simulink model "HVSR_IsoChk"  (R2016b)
settings: Solver=VariableStepAuto  StartTime=0.0  StopTime=10.0  RelTol=1e-3
undefined symbols (not defined in the file or in its folder): bin2dec, enmActv, enmBmsMode, enmCctErr, enmSWSta, HVSR_bIsoResShieldCal, HVSR_bSw1EnaByMnl_C, HVSR_bSw2EnaByMnl_C, HVSR_bSw3EnaByMnl_C, HVSR_bSwEnaByMnl_C, HVSR_bVldEnaByMnl_C, HVSR_cntIsoChkCnfDiag_C, HVSR_cntIsoChkCnfLv1Diag_C, HVSR_cntIsoChkDiag_CW, HVSR_cntPwrDown_C, HVSR_cofPosVoltfilter_C, HVSR_cofResGain_C, HVSR_deltInsRes_C, HVSR_InsResCtrlSw_C, HVSR_kSlopeVal_C, HVSR_numBgnTimeCnt_C, HVSR_numCycleTimeCnt_C, HVSR_numIsoCnst_C, HVSR_numSlopeCnfrm_C, HVSR_ResFirstCtrlSw_C, HVSR_resIsoFaultLvl1Thres_C, HVSR_resIsoFaultLvl2Thres_C, HVSR_ResR1_C, HVSR_ResR2_C, HVSR_ResR3_C, HVSR_resRstnUpLim_C, HVSR_rIsoCnfHysDiag_C, HVSR_rIsoCnfHysLv1Diag_C, HVSR_stBMSModeLvl_C, HVSR_tiChkFilteTime_C, HVSR_tiIsoChkCycl_T, HVSR_tiIsoChkDebounce_C, HVSR_tiIsoVldChkDebounce_C, HVSR_tiTaskTime_C, HVSR_tiVoltDiffThres_C, HVSR_uBattVoltRngHi_C, HVSR_uBattVoltRngLo_C, HVSR_uIsoKVoltThres_C, HVSR_uIsoPosVoltFilter_C, HVSR_uIsoVoltThres_C
libraries: simulink x78
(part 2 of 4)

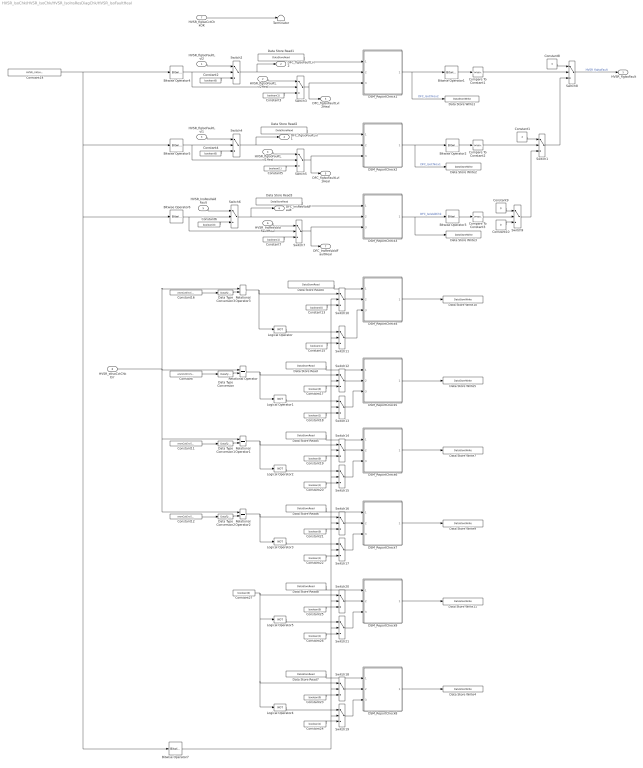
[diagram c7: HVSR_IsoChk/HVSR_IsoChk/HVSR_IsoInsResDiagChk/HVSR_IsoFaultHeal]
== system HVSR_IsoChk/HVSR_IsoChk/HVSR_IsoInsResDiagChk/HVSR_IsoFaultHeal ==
  HVSR_flgIsoFaultLvl2 : Inport
  HVSR_flgIsoFaultLvl2Heal : Inport  Port=2
  HVSR_flgIsoFaultLvl1 : Inport  Port=3
  HVSR_flgIsoFaultLvl1Heal : Inport  Port=4
  HVSR_InsResValdFault : Inport  Port=5
  HVSR_InsResValdFaultHeal : Inport  Port=6
  HVSR_flgIsoCctChkOK : Inport  Port=7
  HVSR_stIsoCctChkErr : Inport  Port=8
  Bitwise Operator1 : simulink/Logic and Bit Operations/Bitwise Operator  logicop=AND  UseBitMask=on  BitMask=bin2dec('00011000')  BitMaskRealWorld=Stored Integer
  Bitwise Operator2 : simulink/Logic and Bit Operations/Bitwise Operator  logicop=AND  UseBitMask=on  BitMask=bin2dec('00011000')  BitMaskRealWorld=Stored Integer
  Bitwise Operator3 : simulink/Logic and Bit Operations/Bitwise Operator  logicop=AND  UseBitMask=on  BitMask=bin2dec('00011000')  BitMaskRealWorld=Stored Integer
  Bitwise Operator4 : simulink/Logic and Bit Operations/Bitwise Operator  logicop=AND  UseBitMask=on  BitMask=bin2dec('00000001')  BitMaskRealWorld=Stored Integer
  Bitwise Operator5 : simulink/Logic and Bit Operations/Bitwise Operator  logicop=AND  UseBitMask=on  BitMask=bin2dec('00000010')  BitMaskRealWorld=Stored Integer
  Bitwise Operator6 : simulink/Logic and Bit Operations/Bitwise Operator  logicop=AND  UseBitMask=on  BitMask=bin2dec('00000100')  BitMaskRealWorld=Stored Integer
  Bitwise Operator7 : simulink/Logic and Bit Operations/Bitwise Operator  logicop=AND  UseBitMask=on  BitMask=bin2dec('00001000')  BitMaskRealWorld=Stored Integer
  Compare To Constant1 : simulink/Logic and Bit Operations/Compare To Constant  relop===  const=24  OutDataTypeStr=boolean
  Compare To Constant2 : simulink/Logic and Bit Operations/Compare To Constant  relop===  const=24  OutDataTypeStr=boolean
  Compare To Constant3 : simulink/Logic and Bit Operations/Compare To Constant  relop===  const=24  OutDataTypeStr=boolean
  Constant : Constant  Value=enmCctErr.S1ERR  OutDataTypeStr=Enum: enmCctErr
  Constant1 : Constant  Value=2  OutDataTypeStr=uint8
  Constant10 : Constant  Value=0  OutDataTypeStr=uint8
  Constant11 : Constant  Value=enmCctErr.S2ERR  OutDataTypeStr=Enum: enmCctErr
  Constant12 : Constant  Value=enmCctErr.S3ERR  OutDataTypeStr=Enum: enmCctErr
  Constant{2,4,6,13,17,19,21,23,25,27} (10 alike) : Constant  Value=boolean(0)
  Constant14 : Constant  Value=HVSR_cntIsoChkDiag_CW
  Constant{3,5,7,15,18,20,22,24,26} (9 alike) : Constant  Value=boolean(1)
  Constant16 : Constant  Value=enmCctErr.CCTCLS  OutDataTypeStr=Enum: enmCctErr
  Constant8 : Constant  Value=3  OutDataTypeStr=uint8
  Constant9 : Constant  Value=0  OutDataTypeStr=uint8
  DSM_ReportCheck1 : Subsystem  TreatAsAtomicUnit=on  RTWFcnName=DSM_ReportCheck  RTWFileName=SrvLib
  DSM_ReportCheck2 : Subsystem  TreatAsAtomicUnit=on  RTWFcnName=DSM_ReportCheck  RTWFileName=SrvLib
  DSM_ReportCheck3 : Subsystem  TreatAsAtomicUnit=on  RTWFcnName=DSM_ReportCheck  RTWFileName=SrvLib
  DSM_ReportCheck4 : Subsystem  TreatAsAtomicUnit=on  RTWFcnName=DSM_ReportCheck  RTWFileName=SrvLib
  DSM_ReportCheck5 : Subsystem  TreatAsAtomicUnit=on  RTWFcnName=DSM_ReportCheck  RTWFileName=SrvLib
  DSM_ReportCheck6 : Subsystem  TreatAsAtomicUnit=on  RTWFcnName=DSM_ReportCheck  RTWFileName=SrvLib
  DSM_ReportCheck7 : Subsystem  TreatAsAtomicUnit=on  RTWFcnName=DSM_ReportCheck  RTWFileName=SrvLib
  DSM_ReportCheck8 : Subsystem  TreatAsAtomicUnit=on  RTWFcnName=DSM_ReportCheck  RTWFileName=SrvLib
  DSM_ReportCheck9 : Subsystem  TreatAsAtomicUnit=on  RTWFcnName=DSM_ReportCheck  RTWFileName=SrvLib
  Data Store Read : DataStoreRead  DataStoreName=DFC_IsoS1SwStuckOpen
  Data Store Read1 : DataStoreRead  DataStoreName=DFC_IsoChkLv2
  Data Store Read2 : DataStoreRead  DataStoreName=DFC_IsoChkLv1
  Data Store Read3 : DataStoreRead  DataStoreName=DFC_InsResValdFault
  Data Store Read4 : DataStoreRead  DataStoreName=DFC_IsoS3SwStuckClsd
  Data Store Read5 : DataStoreRead  DataStoreName=DFC_IsoS2SwStuckOpen
  Data Store Read6 : DataStoreRead  DataStoreName=DFC_IsoS3SwStuckOpen
  Data Store Read7 : DataStoreRead  DataStoreName=DFC_IsoS1SwStuckClsd
  Data Store Read8 : DataStoreRead  DataStoreName=DFC_IsoS2SwStuckClsd
  Data Store Write1 : DataStoreWrite  DataStoreName=DFC_IsoChkLv2
  Data Store Write10 : DataStoreWrite  DataStoreName=DFC_IsoS3SwStuckClsd
  Data Store Write11 : DataStoreWrite  DataStoreName=DFC_IsoS2SwStuckClsd
  Data Store Write2 : DataStoreWrite  DataStoreName=DFC_IsoChkLv1
  Data Store Write3 : DataStoreWrite  DataStoreName=DFC_InsResValdFault
  Data Store Write4 : DataStoreWrite  DataStoreName=DFC_IsoS1SwStuckClsd
  Data Store Write5 : DataStoreWrite  DataStoreName=DFC_IsoS1SwStuckOpen
  Data Store Write7 : DataStoreWrite  DataStoreName=DFC_IsoS2SwStuckOpen
  Data Store Write9 : DataStoreWrite  DataStoreName=DFC_IsoS3SwStuckOpen
  Data Type Conversion{,1..3} (4 alike) : DataTypeConversion  OutDataTypeStr=uint8
  Logical Operator{,1..5} (6 alike) : Logic  Operator=NOT  AllPortsSameDT=off  OutDataTypeStr=boolean
  Relational Operator{,1..3} (4 alike) : RelationalOperator  Operator===  OutDataTypeStr=boolean  RndMeth=Simplest
  Switch{1..21} (21 alike) : Switch  Criteria=u2 ~= 0
  Terminator : Terminator
  " HVSR_flgIsoFault" : Outport
  DFC_flgIsoFaultLvl2 : Outport  Port=2
  DFC_flgIsoFaultLvl2Heal : Outport  Port=3
  DFC_flgIsoFaultLvl1 : Outport  Port=4
  DFC_flgIsoFaultLvl1Heal : Outport  Port=5
  DFC_InsResValdFault : Outport  Port=6
  DFC_InsResValdFaultHeal : Outport  Port=7
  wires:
  Constant14/1 -> Bitwise Operator4/1, Bitwise Operator5/1, Bitwise Operator6/1, Bitwise Operator7/1
  DSM_ReportCheck1/1(Dfc_id) -> Data Store Write1/1, Bitwise Operator1/1  "DFC_IsoChkLv2"
  DSM_ReportCheck2/1(Dfc_id) -> Data Store Write2/1, Bitwise Operator2/1  "DFC_IsoChkLv1"
  Bitwise Operator2/1 -> Compare To Constant2/1
  Bitwise Operator1/1 -> Compare To Constant1/1
  DSM_ReportCheck3/1(Dfc_id) -> Bitwise Operator3/1, Data Store Write3/1  "DFC_IsoValdChk"
  Data Store Read2/1 -> DSM_ReportCheck2/1(Dfc_id_nv)
  Switch8/1 -> " HVSR_flgIsoFault"/1  "HVSR_flgIsoFault"
  Data Store Read3/1 -> DSM_ReportCheck3/1(Dfc_id_nv)
  Data Store Read1/1 -> DSM_ReportCheck1/1(Dfc_id_nv)
  Switch6/1 -> DFC_InsResValdFault/1, DSM_ReportCheck3/2(Err)
  Switch4/1 -> DFC_flgIsoFaultLvl1/1, DSM_ReportCheck2/2(Err)
  Switch3/1 -> DFC_flgIsoFaultLvl2Heal/1, DSM_ReportCheck1/3(Heal)
  Switch2/1 -> DFC_flgIsoFaultLvl2/1, DSM_ReportCheck1/2(Err)
  Switch7/1 -> DFC_InsResValdFaultHeal/1, DSM_ReportCheck3/3(Heal)
  Switch5/1 -> DFC_flgIsoFaultLvl1Heal/1, DSM_ReportCheck2/3(Heal)
  Constant2/1 -> Switch2/3
  Bitwise Operator4/1 -> Switch3/2, Switch2/2
  HVSR_flgIsoFaultLvl2/1 -> Switch2/1
  Constant3/1 -> Switch3/3
  HVSR_flgIsoFaultLvl2Heal/1 -> Switch3/1
  Constant4/1 -> Switch4/3
  Constant5/1 -> Switch5/3
  HVSR_flgIsoFaultLvl1/1 -> Switch4/1
  Bitwise Operator5/1 -> Switch5/2, Switch4/2
  HVSR_flgIsoFaultLvl1Heal/1 -> Switch5/1
  Constant6/1 -> Switch6/3
  Bitwise Operator6/1 -> Switch7/2, Switch6/2
  HVSR_InsResValdFault/1 -> Switch6/1
  Constant7/1 -> Switch7/3
  HVSR_InsResValdFaultHeal/1 -> Switch7/1
  Compare To Constant1/1 -> Switch8/2
  Compare To Constant2/1 -> Switch1/2
  Switch9/1 -> Switch1/3
  Constant1/1 -> Switch1/1
  Constant8/1 -> Switch8/1
  Switch1/1 -> Switch8/3
  Bitwise Operator3/1 -> Compare To Constant3/1
  Compare To Constant3/1 -> Switch9/2
  Constant9/1 -> Switch9/1
  Constant10/1 -> Switch9/3
  DSM_ReportCheck4/1(Dfc_id) -> Data Store Write10/1
  Data Store Read4/1 -> DSM_ReportCheck4/1(Dfc_id_nv)
  Relational Operator3/1 -> Logical Operator/1, Switch10/1
  Constant13/1 -> Switch10/3
  Constant15/1 -> Switch11/3
  Logical Operator/1 -> Switch11/1
  Switch11/1 -> DSM_ReportCheck4/3(Heal)
  Switch10/1 -> DSM_ReportCheck4/2(Err)
  Constant/1 -> Data Type Conversion/1
  Data Type Conversion/1 -> Relational Operator/2
  Constant11/1 -> Data Type Conversion1/1
  Data Type Conversion1/1 -> Relational Operator1/2
  Constant12/1 -> Data Type Conversion2/1
  Data Type Conversion2/1 -> Relational Operator2/2
  HVSR_stIsoCctChkErr/1 -> Relational Operator3/1, Relational Operator2/1, Relational Operator1/1, Relational Operator/1
  Constant16/1 -> Data Type Conversion3/1
  Data Type Conversion3/1 -> Relational Operator3/2
  DSM_ReportCheck5/1(Dfc_id) -> Data Store Write5/1
  Data Store Read/1 -> DSM_ReportCheck5/1(Dfc_id_nv)
  Switch12/1 -> DSM_ReportCheck5/2(Err)
  Relational Operator/1 -> Logical Operator1/1, Switch12/1
  Constant17/1 -> Switch12/3
  Switch13/1 -> DSM_ReportCheck5/3(Heal)
  Logical Operator1/1 -> Switch13/1
  Constant18/1 -> Switch13/3
  DSM_ReportCheck6/1(Dfc_id) -> Data Store Write7/1
  Data Store Read5/1 -> DSM_ReportCheck6/1(Dfc_id_nv)
  Switch14/1 -> DSM_ReportCheck6/2(Err)
  Relational Operator1/1 -> Logical Operator2/1, Switch14/1
  Constant19/1 -> Switch14/3
  Switch15/1 -> DSM_ReportCheck6/3(Heal)
  Logical Operator2/1 -> Switch15/1
  DSM_ReportCheck7/1(Dfc_id) -> Data Store Write9/1
  Data Store Read6/1 -> DSM_ReportCheck7/1(Dfc_id_nv)
  Switch16/1 -> DSM_ReportCheck7/2(Err)
  Relational Operator2/1 -> Logical Operator3/1, Switch16/1
  Constant21/1 -> Switch16/3
  Switch17/1 -> DSM_ReportCheck7/3(Heal)
  Logical Operator3/1 -> Switch17/1
  Constant20/1 -> Switch15/3
  Constant22/1 -> Switch17/3
  HVSR_flgIsoCctChkOK/1 -> Terminator/1
  DSM_ReportCheck8/1(Dfc_id) -> Data Store Write4/1
  Data Store Read7/1 -> DSM_ReportCheck8/1(Dfc_id_nv)
  Switch18/1 -> DSM_ReportCheck8/2(Err)
  Constant27/1 -> Switch18/1, Logical Operator4/1, Logical Operator5/1, Switch20/1
  Constant23/1 -> Switch18/3
  Switch19/1 -> DSM_ReportCheck8/3(Heal)
  Logical Operator4/1 -> Switch19/1
  Constant24/1 -> Switch19/3
  DSM_ReportCheck9/1(Dfc_id) -> Data Store Write11/1
  Data Store Read8/1 -> DSM_ReportCheck9/1(Dfc_id_nv)
  Switch20/1 -> DSM_ReportCheck9/2(Err)
  Constant25/1 -> Switch20/3
  Switch21/1 -> DSM_ReportCheck9/3(Heal)
  Logical Operator5/1 -> Switch21/1
  Constant26/1 -> Switch21/3
  Bitwise Operator7/1 -> Switch19/2, Switch18/2, Switch21/2, Switch20/2, Switch17/2, Switch16/2, Switch15/2, Switch14/2, Switch13/2, Switch12/2, Switch10/2, Switch11/2

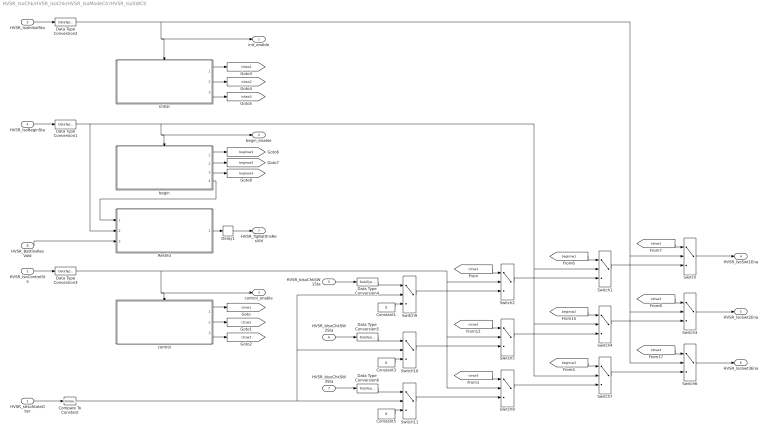
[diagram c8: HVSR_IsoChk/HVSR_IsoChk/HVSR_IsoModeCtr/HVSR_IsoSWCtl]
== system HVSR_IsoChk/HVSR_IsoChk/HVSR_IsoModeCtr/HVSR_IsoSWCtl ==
  HVSR_stIsoStateObsr : Inport
  HVSR_IsoControlSta : Inport  Port=2
  HVSR_IsoInitialSta : Inport  Port=3
  HVSR_IsoBeginSta : Inport  Port=4
  HVSR_bIsoChkSW1Sta : Inport  Port=5
  HVSR_bIsoChkSW2Sta : Inport  Port=6
  HVSR_bIsoChkSW3Sta : Inport  Port=7
  HVSR_BattInsResVald : Inport  Port=8
  Compare To Constant : simulink/Logic and Bit Operations/Compare To Constant  relop===  const=8  OutDataTypeStr=boolean
  Constant1 : Constant  Value=0  OutDataTypeStr=boolean
  Constant3 : Constant  Value=0  OutDataTypeStr=boolean
  Constant5 : Constant  Value=0  OutDataTypeStr=boolean
  Data Type Conversion{1..6} (6 alike) : DataTypeConversion  OutDataTypeStr=boolean
  Delay1 : Delay  DelayLength=1  InitialCondition=0
  Initial : Subsystem  Description=Battery pack insulation detection initialization module  TreatAsAtomicUnit=on
  ResVld : Subsystem
  Switch{,1..11} (12 alike) : Switch  Criteria=u2 ~= 0
  begin : Subsystem  Description=Battery pack insulation detection initialization module  TreatAsAtomicUnit=on
  control : Subsystem  Description=Battery pack insulation detection initialization module  TreatAsAtomicUnit=on
  init_enable : Outport
  begin_enable : Outport  Port=2
  control_enable : Outport  Port=3
  HVSR_IsoSwt1Ena : Outport  Port=4
  HVSR_IsoSwt2Ena : Outport  Port=5
  HVSR_IsoSwt3Ena : Outport  Port=6
  HVSR_flgBattInsResVld : Outport  Port=7
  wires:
  ResVld/1(HVSR_flgBattInsResVld) -> Delay1/1
  Delay1/1 -> HVSR_flgBattInsResVld/1
  HVSR_BattInsResVald/1 -> ResVld/3(HVSR_BattInsResVald)
  begin/4(reset_flgVald) -> ResVld/1(reset_flgVald)
  HVSR_IsoInitialSta/1 -> Data Type Conversion2/1
  HVSR_IsoBeginSta/1 -> Data Type Conversion1/1
  HVSR_IsoControlSta/1 -> Data Type Conversion3/1
  control/1(ctr_bIsoSwt1Ena) -> [ctrsw1]
  control/3(ctr_bIsoSwt3Ena) -> [ctrsw3]
  control/2(ctr_bIsoSwt2Ena) -> [ctrsw2]
  Initial/1(init_bIsoSwt1Ena) -> [initsw1]
  Initial/2(init_bIsoSwt2Ena) -> [initsw2]
  Initial/3(init_bIsoSwt3Ena) -> [initsw3]
  begin/1(begin_bIsoSwt1Ena) -> [beginsw1]
  begin/2(begin_bIsoSwt2Ena) -> [beginsw2]
  begin/3(begin_bIsoSwt3Ena) -> [beginsw3]
  Switch/1 -> HVSR_IsoSwt1Ena/1
  Switch1/1 -> Switch/3
  [beginsw1] -> Switch1/1
  [ctrsw1] -> Switch2/1
  Switch9/1 -> Switch2/3
  [initsw1] -> Switch/1
  Switch2/1 -> Switch1/3
  Switch3/1 -> HVSR_IsoSwt2Ena/1
  Switch4/1 -> Switch3/3
  [beginsw2] -> Switch4/1
  [ctrsw2] -> Switch5/1
  Switch10/1 -> Switch5/3
  [initsw2] -> Switch3/1
  Switch5/1 -> Switch4/3
  Switch6/1 -> HVSR_IsoSwt3Ena/1
  Data Type Conversion2/1 -> init_enable/1, Initial/Enable, Switch6/2, Switch3/2, Switch/2
  Switch7/1 -> Switch6/3
  Data Type Conversion1/1 -> ResVld/2(HVSR_IsoBeginSta), begin_enable/1, begin/Enable, Switch7/2, Switch4/2, Switch1/2
  [beginsw3] -> Switch7/1
  Data Type Conversion3/1 -> Switch8/2, Switch5/2, Switch2/2, control_enable/1, control/Enable
  [ctrsw3] -> Switch8/1
  [initsw3] -> Switch6/1
  Switch8/1 -> Switch7/3
  Switch11/1 -> Switch8/3
  Data Type Conversion4/1 -> Switch9/1
  Constant1/1 -> Switch9/3
  Data Type Conversion5/1 -> Switch10/1
  Constant3/1 -> Switch10/3
  Compare To Constant/1 -> Switch11/2, Switch10/2, Switch9/2
  Data Type Conversion6/1 -> Switch11/1
  Constant5/1 -> Switch11/3
  HVSR_stIsoStateObsr/1 -> Compare To Constant/1
  HVSR_bIsoChkSW1Sta/1 -> Data Type Conversion4/1
  HVSR_bIsoChkSW2Sta/1 -> Data Type Conversion5/1
  HVSR_bIsoChkSW3Sta/1 -> Data Type Conversion6/1

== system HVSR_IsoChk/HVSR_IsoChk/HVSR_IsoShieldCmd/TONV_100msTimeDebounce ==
  note: Turn On Delay Time Deboune
  u : Inport
  T : Inport  Port=2
  Add : Sum
  Constant1 : Constant  Value=0  OutDataTypeStr=single
  Constant2 : Constant  OutDataTypeStr=uint8
  Constant3 : Constant  Value=0  OutDataTypeStr=uint8
  Constant4 : Constant  Value=0.1  OutDataTypeStr=single
  Delay : Delay  DelayLength=1  InitialCondition=0
  MinMax : MinMax  Inputs=2
  Product : Product  OutMin=[0]  OutMax=[65535]  OutDataTypeStr=single
  Relational Operator : RelationalOperator  Operator=>  OutDataTypeStr=boolean  RndMeth=Simplest
  Switch : Switch  Criteria=u2 ~= 0
  Switch1 : Switch  Criteria=u2 ~= 0
  y : Outport
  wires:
  Switch1/1 -> Product/1
  Constant3/1 -> Switch1/3
  Constant2/1 -> Switch1/1
  u/1 -> Switch1/2, Switch/2
  Constant4/1 -> Switch/1
  Constant1/1 -> Switch/3
  Add/1 -> Product/2
  Product/1 -> Relational Operator/1, Delay/1
  Switch/1 -> Add/1
  Delay/1 -> MinMax/2
  Relational Operator/1 -> y/1
  T/1 -> MinMax/1, Relational Operator/2
  MinMax/1 -> Add/2

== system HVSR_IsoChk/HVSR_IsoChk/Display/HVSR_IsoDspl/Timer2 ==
  En : Inport
  Ts : Inport  Port=2
  Add : Sum
  Constant5 : Constant  Value=single(0)  OutDataTypeStr=single
  Switch2 : Switch  Criteria=u2 ~= 0
  Unit Delay : UnitDelay  SampleTime=-1
  Timer : Outport
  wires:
  Unit Delay/1 -> Add/2
  En/1 -> Switch2/2
  Ts/1 -> Switch2/1
  Constant5/1 -> Switch2/3
  Switch2/1 -> Add/1
  Add/1 -> Timer/1, Unit Delay/1  "HVSR_tiIsoChkTimer"

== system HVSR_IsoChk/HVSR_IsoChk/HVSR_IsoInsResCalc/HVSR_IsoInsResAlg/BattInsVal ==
  HVSR_flgInsResVld : Inport
  HVSR_resBattInsRes : Inport  Port=2
  HVSR_resIsoTheory : Inport  Port=3
  Constant1 : Constant  Value=HVSR_InsResCtrlSw_C
  Delay : Delay  DelayLength=1  InitialCondition=0
  Delay1 : Delay  DelayLength=1  InitialCondition=0
  HVSR_IsoInsShkFilter : Subsystem
  Logical Operator : Logic  AllPortsSameDT=off  OutDataTypeStr=boolean
  Subsystem1 : Subsystem
  Switch : Switch  Criteria=u2 ~= 0
  Switch1 : Switch  Criteria=u2 ~= 0
  HVSR_IsoBattInsRes : Outport
  HVSR_IsoInsResTheory : Outport  Port=2
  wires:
  HVSR_flgInsResVld/1 -> Logical Operator/1, HVSR_IsoInsShkFilter/1(HVSR_flgInsResVld)
  HVSR_resIsoTheory/1 -> Switch1/3, Delay1/1
  HVSR_resBattInsRes/1 -> Switch/3, Delay/1, HVSR_IsoInsShkFilter/2(HVSR_resBattInsRes)
  Delay/1 -> Subsystem1/1(InsRes)
  Delay1/1 -> Subsystem1/2(InsTheory)
  Switch/1 -> HVSR_IsoBattInsRes/1
  HVSR_IsoInsShkFilter/1(HVSR_flgInsResChngVld) -> Logical Operator/2
  Logical Operator/1 -> Subsystem1/Trigger  "HVSR_flgIsoVldLmt"
  Subsystem1/1(BattInsRes) -> Switch/1
  Subsystem1/2(HVSR_resIsoTheory) -> Switch1/1
  Switch1/1 -> HVSR_IsoInsResTheory/1
  Constant1/1 -> Switch/2, Switch1/2

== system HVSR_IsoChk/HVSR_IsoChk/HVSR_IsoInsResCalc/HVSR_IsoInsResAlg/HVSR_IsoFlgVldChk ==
  IsoSwtLastTEna : Inport
  HVSR_uScndRsVlot : Inport  Port=2
  HVSR_flgScndRsVlotVld : Inport  Port=3
  HVSR_uBattVolt : Inport  Port=4
  HVSR_uFrstRsVlot : Inport  Port=5
  HVSR_flgFrstRsVlotVld : Inport  Port=6
  begin_enable : Inport  Port=7
  control_enable : Inport  Port=8
  Constant1 : Constant  OutDataTypeStr=boolean
  HVSR_IsoFlgResVld : Subsystem  TreatAsAtomicUnit=on
  HVSR_IsoParVldChk : Subsystem
  HVSR_flgInsResVld : Outport
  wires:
  control_enable/1 -> HVSR_IsoFlgResVld/3(control_enable)
  begin_enable/1 -> HVSR_IsoFlgResVld/2(begin_enable)
  HVSR_uBattVolt/1 -> HVSR_IsoFlgResVld/1(BSPR_uBattVolt)
  HVSR_flgScndRsVlotVld/1 -> HVSR_IsoFlgResVld/7(HVSR_flgScndRsVlotVld), HVSR_IsoParVldChk/5(HVSR_flgScndRsVlotVld)
  HVSR_uScndRsVlot/1 -> HVSR_IsoFlgResVld/6(HVSR_uScndRsVlot), HVSR_IsoParVldChk/4(HVSR_uScndRsVlot)
  HVSR_uFrstRsVlot/1 -> HVSR_IsoParVldChk/2(HVSR_uFrstRsVlot), HVSR_IsoFlgResVld/4(HVSR_uFrstRsVlot)
  HVSR_flgFrstRsVlotVld/1 -> HVSR_IsoFlgResVld/5(HVSR_flgFrstRsVlotVld), HVSR_IsoParVldChk/3(HVSR_flgFrstRsVlotVld)
  HVSR_IsoFlgResVld/1(HVSR_flgBattInsResVld) -> HVSR_IsoParVldChk/1(HVSR_flgBattInsResVld)
  Constant1/1 -> HVSR_IsoParVldChk/6(In6)
  IsoSwtLastTEna/1 -> HVSR_IsoParVldChk/7(IsoSwtLastTEna)
  HVSR_IsoParVldChk/1(HVSR_flgInsResVld) -> HVSR_flgInsResVld/1

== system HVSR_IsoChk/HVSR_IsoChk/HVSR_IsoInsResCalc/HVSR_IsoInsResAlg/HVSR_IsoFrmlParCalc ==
  note: 10
  note: 0.1s
  note: 2V/0.1s=20
  begin_on : Inport
  control_on : Inport  Port=2
  HVSR_uIsoRsVolt : Inport  Port=3
  BSPR_uBattVolt : Inport  Port=4
  Constant : Constant  Value=HVSR_kSlopeVal_C
  Constant1 : Constant  Value=HVSR_tiIsoChkCycl_T
  Constant2 : Constant  Value=HVSR_numSlopeCnfrm_C  VectorParams1D=off
  HVSR_IsoαCalc : Subsystem  Description=Stores the voltage value of the power battery to the body shell after closing the relay  TreatAsAtomicUnit=on
  HVSR_IsoβCalc : Subsystem  Description=Stores the voltage value of the power battery to the body shell after closing the relay  TreatAsAtomicUnit=on
  HVSR_uBattVoltFilter : Subsystem  Description=Stores the voltage value of the power battery to the body shell after closing the relay  TreatAsAtomicUnit=on
  HVSR_uIsoScndRsVolt : Outport
  HVSR_uScndRsVlot : Outport  Port=2  InitialOutput=0
  HVSR_flgScndRsVlotVld : Outport  Port=3
  HVSR_uBattVolt : Outport  Port=4
  HVSR_uIsoFrstRsVolt : Outport  Port=5
  HVSR_uFrstRsVlot : Outport  Port=6  InitialOutput=0
  HVSR_flgFrstRsVlotVld : Outport  Port=7
  HVSR_numIsoFrstVal : Outport  Port=8
  HVSR_numIsoScndVal : Outport  Port=9
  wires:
  HVSR_IsoαCalc/1(HVSR_uIsoFrstRsVolt) -> HVSR_uIsoFrstRsVolt/1  "HVSR_uIsoFrstRsVolt"
  HVSR_uIsoRsVolt/1 -> HVSR_IsoαCalc/1(HVSR_uIsoRsVolt), HVSR_IsoβCalc/1(HVSR_uIsoRsVolt)
  HVSR_uBattVoltFilter/1(HVSR_uBattVolt) -> HVSR_uBattVolt/1  "HVSR_uBattFilterEnd"
  BSPR_uBattVolt/1 -> HVSR_uBattVoltFilter/1(BSPR_uBattVolt), HVSR_IsoαCalc/5(BSPR_uBattVolt), HVSR_IsoβCalc/5(BSPR_uBattVolt)
  begin_on/1 -> HVSR_IsoαCalc/Action
  HVSR_IsoαCalc/4(HVSR_numIsoFrstVal) -> HVSR_numIsoFrstVal/1  "HVSR_numIsoFrstVal"
  HVSR_IsoβCalc/1(HVSR_uIsoScndRsVolt) -> HVSR_uIsoScndRsVolt/1  "HVSR_uIsoScndRsVolt"
  control_on/1 -> HVSR_IsoβCalc/Action
  HVSR_IsoαCalc/2(HVSR_uFrstRsVlot) -> HVSR_uFrstRsVlot/1  "HVSR_uFrstRsVlot"
  HVSR_IsoβCalc/2(HVSR_uScndRsVlot) -> HVSR_uScndRsVlot/1  "HVSR_uScndRsVlot"
  HVSR_IsoαCalc/3(HVSR_flgFrstRsVlotVld) -> HVSR_flgFrstRsVlotVld/1  "HVSR_flgFrstRsVlotVld"
  HVSR_IsoβCalc/4(HVSR_numIsoScndVal) -> HVSR_numIsoScndVal/1  "HVSR_numIsoScndVal"
  HVSR_IsoβCalc/3(HVSR_flgScndRsVlotVld) -> HVSR_flgScndRsVlotVld/1  "HVSR_flgScndRsVlotVld"
  Constant/1 -> HVSR_IsoαCalc/2(HVSR_kSlopeVal), HVSR_IsoβCalc/2(HVSR_kSlopeVal)
  Constant1/1 -> HVSR_IsoαCalc/3(HVSR_tiIsoChkCycl_T), HVSR_IsoβCalc/3(HVSR_tiIsoChkCycl_T)
  Constant2/1 -> HVSR_IsoαCalc/4(HVSR_numSlopeCnfrm), HVSR_IsoβCalc/4(HVSR_numSlopeCnfrm)

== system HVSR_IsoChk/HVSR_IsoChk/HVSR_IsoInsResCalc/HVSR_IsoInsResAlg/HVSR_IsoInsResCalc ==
  HVSR_numIsoFrstVal : Inport
  HVSR_numIsoScndVal : Inport  Port=2
  Enable : EnablePort
  HVSR_IsoBattNegInsRes : Subsystem  Description=When the input negative voltage is higher than the positive voltage, calculate the insulation resistance value  TreatAsAtomicUnit=on
  HVSR_IsoBattPosInsRes : Subsystem  Description=When the input negative voltage is higher than the positive voltage, calculate the insulation resistance value  TreatAsAtomicUnit=on
  MinMax : MinMax  Inputs=2
  R0 : Subsystem
  Subsystem : Subsystem  Commented=through
  HVSR_resBattInsRes : Outport
  HVSR_resIsoTheory : Outport  Port=2
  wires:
  Subsystem/1(HVSR_resIsoTheory) -> HVSR_resIsoTheory/1
  R0/1(HVSR_ResR0_C) -> HVSR_IsoBattNegInsRes/3(HVSR_ResR0_C), HVSR_IsoBattPosInsRes/3(HVSR_ResR0_C)
  HVSR_numIsoFrstVal/1 -> HVSR_IsoBattNegInsRes/1(Numα), HVSR_IsoBattPosInsRes/1(Numα)
  HVSR_numIsoScndVal/1 -> HVSR_IsoBattNegInsRes/2(Numβ), HVSR_IsoBattPosInsRes/2(Numβ)
  MinMax/1 -> HVSR_resBattInsRes/1, Subsystem/1(Rp')
  HVSR_IsoBattNegInsRes/1(HVSR_resBattInsRes) -> MinMax/1  "HVSR_resBattInsRes1"
  HVSR_IsoBattPosInsRes/1(HVSR_resBattInsRes) -> MinMax/2  "HVSR_resBattInsRes2"

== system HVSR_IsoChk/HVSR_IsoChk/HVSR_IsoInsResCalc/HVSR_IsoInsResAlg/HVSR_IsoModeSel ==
  begin_enable : Inport
  control_enable : Inport  Port=2
  If : If  NumInputs=2  IfExpression=(u1 == 1)&(u2 ~= 1)  ElseIfExpressions=(u1 ~= 1)&(u2 == 1)
  begin_on : Outport
  Out3 : Outport  Port=2
  control_on : Outport  Port=3
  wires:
  begin_enable/1 -> If/1
  control_enable/1 -> If/2
  If/2 -> control_on/1
  If/1 -> begin_on/1
  If/3 -> Out3/1

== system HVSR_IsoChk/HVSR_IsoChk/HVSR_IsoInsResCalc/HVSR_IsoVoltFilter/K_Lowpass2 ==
  k : Inport
  u : Inport  Port=2
  Add : Sum
  Constant2 : Constant  Value=0  OutDataTypeStr=boolean
  Delay : Delay  DelayLength=1  InitialCondition=1
  Product : Product
  Subtract : Sum  Inputs=+-
  Switch1 : Switch  Criteria=u2 > Threshold
  Unit Delay : UnitDelay  SampleTime=-1
  y : Outport
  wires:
  k/1 -> Product/1
  Product/1 -> Add/1
  Constant2/1 -> Delay/1
  Unit Delay/1 -> Subtract/2, Add/2
  Subtract/1 -> Product/2
  Add/1 -> Switch1/3
  Delay/1 -> Switch1/2
  Switch1/1 -> y/1, Unit Delay/1
  u/1 -> Switch1/1, Subtract/1

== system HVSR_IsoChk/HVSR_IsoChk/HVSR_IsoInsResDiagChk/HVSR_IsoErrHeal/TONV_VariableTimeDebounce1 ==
  note: Turn On Delay Time Deboune
  u : Inport
  T : Inport  Port=2
  dT : Inport  Port=3
  Add : Sum
  Constant1 : Constant  Value=0  OutDataTypeStr=single
  Constant2 : Constant  OutDataTypeStr=uint8
  Constant3 : Constant  Value=0  OutDataTypeStr=uint8
  Delay : Delay  DelayLength=1  InitialCondition=0
  MinMax : MinMax  Inputs=2
  Product : Product  OutMin=[0]  OutMax=[65535]  OutDataTypeStr=single
  Relational Operator : RelationalOperator  Operator=>  OutDataTypeStr=boolean  RndMeth=Simplest
  Switch : Switch  Criteria=u2 ~= 0
  Switch1 : Switch  Criteria=u2 ~= 0
  y : Outport
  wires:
  MinMax/1 -> Add/2
  T/1 -> Relational Operator/2, MinMax/1
  Relational Operator/1 -> y/1
  Delay/1 -> MinMax/2
  Switch/1 -> Add/1
  Product/1 -> Delay/1, Relational Operator/1
  Add/1 -> Product/2
  Constant1/1 -> Switch/3
  dT/1 -> Switch/1
  u/1 -> Switch/2, Switch1/2
  Constant2/1 -> Switch1/1
  Constant3/1 -> Switch1/3
  Switch1/1 -> Product/1

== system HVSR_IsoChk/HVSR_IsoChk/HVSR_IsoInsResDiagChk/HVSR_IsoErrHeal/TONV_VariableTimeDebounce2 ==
  note: Turn On Delay Time Deboune
  u : Inport
  T : Inport  Port=2
  dT : Inport  Port=3
  Add : Sum
  Constant1 : Constant  Value=0  OutDataTypeStr=single
  Constant2 : Constant  OutDataTypeStr=uint8
  Constant3 : Constant  Value=0  OutDataTypeStr=uint8
  Delay : Delay  DelayLength=1  InitialCondition=0
  MinMax : MinMax  Inputs=2
  Product : Product  OutMin=[0]  OutMax=[65535]  OutDataTypeStr=single
  Relational Operator : RelationalOperator  Operator=>  OutDataTypeStr=boolean  RndMeth=Simplest
  Switch : Switch  Criteria=u2 ~= 0
  Switch1 : Switch  Criteria=u2 ~= 0
  y : Outport
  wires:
  Switch1/1 -> Product/1
  Constant3/1 -> Switch1/3
  Constant2/1 -> Switch1/1
  u/1 -> Switch1/2, Switch/2
  dT/1 -> Switch/1
  Constant1/1 -> Switch/3
  Add/1 -> Product/2
  Product/1 -> Relational Operator/1, Delay/1
  Switch/1 -> Add/1
  Delay/1 -> MinMax/2
  Relational Operator/1 -> y/1
  T/1 -> MinMax/1, Relational Operator/2
  MinMax/1 -> Add/2

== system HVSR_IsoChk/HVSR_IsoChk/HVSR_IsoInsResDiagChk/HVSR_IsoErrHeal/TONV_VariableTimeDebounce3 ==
  note: Turn On Delay Time Deboune
  u : Inport
  T : Inport  Port=2
  dT : Inport  Port=3
  Add : Sum
  Constant1 : Constant  Value=0  OutDataTypeStr=single
  Constant2 : Constant  OutDataTypeStr=uint8
  Constant3 : Constant  Value=0  OutDataTypeStr=uint8
  Delay : Delay  DelayLength=1  InitialCondition=0
  MinMax : MinMax  Inputs=2
  Product : Product  OutMin=[0]  OutMax=[65535]  OutDataTypeStr=single
  Relational Operator : RelationalOperator  Operator=>  OutDataTypeStr=boolean  RndMeth=Simplest
  Switch : Switch  Criteria=u2 ~= 0
  Switch1 : Switch  Criteria=u2 ~= 0
  y : Outport
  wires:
  MinMax/1 -> Add/2
  T/1 -> Relational Operator/2, MinMax/1
  Relational Operator/1 -> y/1
  Delay/1 -> MinMax/2
  Switch/1 -> Add/1
  Product/1 -> Delay/1, Relational Operator/1
  Add/1 -> Product/2
  Constant1/1 -> Switch/3
  dT/1 -> Switch/1
  u/1 -> Switch/2, Switch1/2
  Constant2/1 -> Switch1/1
  Constant3/1 -> Switch1/3
  Switch1/1 -> Product/1

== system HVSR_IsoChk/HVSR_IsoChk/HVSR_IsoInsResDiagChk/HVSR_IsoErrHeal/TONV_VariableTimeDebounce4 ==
  note: Turn On Delay Time Deboune
  u : Inport
  T : Inport  Port=2
  dT : Inport  Port=3
  Add : Sum
  Constant1 : Constant  Value=0  OutDataTypeStr=single
  Constant2 : Constant  OutDataTypeStr=uint8
  Constant3 : Constant  Value=0  OutDataTypeStr=uint8
  Delay : Delay  DelayLength=1  InitialCondition=0
  MinMax : MinMax  Inputs=2
  Product : Product  OutMin=[0]  OutMax=[65535]  OutDataTypeStr=single
  Relational Operator : RelationalOperator  Operator=>  OutDataTypeStr=boolean  RndMeth=Simplest
  Switch : Switch  Criteria=u2 ~= 0
  Switch1 : Switch  Criteria=u2 ~= 0
  y : Outport
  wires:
  Switch1/1 -> Product/1
  Constant3/1 -> Switch1/3
  Constant2/1 -> Switch1/1
  u/1 -> Switch1/2, Switch/2
  dT/1 -> Switch/1
  Constant1/1 -> Switch/3
  Add/1 -> Product/2
  Product/1 -> Relational Operator/1, Delay/1
  Switch/1 -> Add/1
  Delay/1 -> MinMax/2
  Relational Operator/1 -> y/1
  T/1 -> MinMax/1, Relational Operator/2
  MinMax/1 -> Add/2

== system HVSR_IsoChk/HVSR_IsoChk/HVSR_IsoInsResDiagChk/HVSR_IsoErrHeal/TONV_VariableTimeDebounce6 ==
  note: Turn On Delay Time Deboune
  u : Inport
  T : Inport  Port=2
  dT : Inport  Port=3
  Add : Sum
  Constant1 : Constant  Value=0  OutDataTypeStr=single
  Constant2 : Constant  OutDataTypeStr=uint8
  Constant3 : Constant  Value=0  OutDataTypeStr=uint8
  Delay : Delay  DelayLength=1  InitialCondition=0
  MinMax : MinMax  Inputs=2
  Product : Product  OutMin=[0]  OutMax=[65535]  OutDataTypeStr=single
  Relational Operator : RelationalOperator  Operator=>  OutDataTypeStr=boolean  RndMeth=Simplest
  Switch : Switch  Criteria=u2 ~= 0
  Switch1 : Switch  Criteria=u2 ~= 0
  y : Outport
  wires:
  MinMax/1 -> Add/2
  T/1 -> Relational Operator/2, MinMax/1
  Relational Operator/1 -> y/1
  Delay/1 -> MinMax/2
  Switch/1 -> Add/1
  Product/1 -> Delay/1, Relational Operator/1
  Add/1 -> Product/2
  Constant1/1 -> Switch/3
  dT/1 -> Switch/1
  u/1 -> Switch/2, Switch1/2
  Constant2/1 -> Switch1/1
  Constant3/1 -> Switch1/3
  Switch1/1 -> Product/1

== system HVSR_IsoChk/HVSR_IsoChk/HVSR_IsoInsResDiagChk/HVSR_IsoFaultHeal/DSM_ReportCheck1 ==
  note: Fault report to diagnostic management system
  Dfc_id_nv : Inport  OutDataTypeStr=uint8
  Err : Inport  Port=2
  Heal : Inport  Port=3
  Bit Clear1 : simulink/Logic and Bit Operations/Bit Clear  iBit=4
  Bit Clear2 : simulink/Logic and Bit Operations/Bit Clear  iBit=3
  Bit Set : simulink/Logic and Bit Operations/Bit Set  iBit=4
  Bit Set1 : simulink/Logic and Bit Operations/Bit Set  iBit=3
  Bit Set2 : simulink/Logic and Bit Operations/Bit Set  iBit=3
  Bit Set4 : simulink/Logic and Bit Operations/Bit Set  iBit=7
  Constant7 : Constant  Value=0  OutDataTypeStr=boolean
  Delay2 : Delay  DelayLength=1  InitialCondition=1
  Delay3 : Delay  DelayLength=1  InitialCondition=0
  Switch2 : Switch  Criteria=u2 ~= 0
  Switch3 : Switch  Criteria=u2 ~= 0
  Switch4 : Switch  Criteria=u2 ~= 0
  Dfc_id : Outport  OutDataTypeStr=uint8
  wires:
  Heal/1 -> Switch4/2
  Delay3/1 -> Switch4/3
  Bit Clear1/1 -> Bit Set2/1
  Bit Set2/1 -> Switch4/1
  Err/1 -> Switch3/2
  Switch4/1 -> Switch3/3
  Bit Set/1 -> Bit Set1/1
  Bit Set1/1 -> Switch3/1
  Switch2/1 -> Dfc_id/1, Delay3/1
  Bit Clear2/1 -> Switch2/1
  Switch3/1 -> Switch2/3
  Delay2/1 -> Switch2/2
  Constant7/1 -> Delay2/1
  Bit Set4/1 -> Bit Set/1
  Dfc_id_nv/1 -> Bit Clear1/1, Bit Set4/1, Bit Clear2/1

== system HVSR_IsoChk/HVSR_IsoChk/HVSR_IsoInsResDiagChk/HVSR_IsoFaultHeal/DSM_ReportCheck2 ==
  note: Fault report to diagnostic management system
  Dfc_id_nv : Inport  OutDataTypeStr=uint8
  Err : Inport  Port=2
  Heal : Inport  Port=3
  Bit Clear1 : simulink/Logic and Bit Operations/Bit Clear  iBit=4
  Bit Clear2 : simulink/Logic and Bit Operations/Bit Clear  iBit=3
  Bit Set : simulink/Logic and Bit Operations/Bit Set  iBit=4
  Bit Set1 : simulink/Logic and Bit Operations/Bit Set  iBit=3
  Bit Set2 : simulink/Logic and Bit Operations/Bit Set  iBit=3
  Bit Set4 : simulink/Logic and Bit Operations/Bit Set  iBit=7
  Constant7 : Constant  Value=0  OutDataTypeStr=boolean
  Delay2 : Delay  DelayLength=1  InitialCondition=1
  Delay3 : Delay  DelayLength=1  InitialCondition=0
  Switch2 : Switch  Criteria=u2 ~= 0
  Switch3 : Switch  Criteria=u2 ~= 0
  Switch4 : Switch  Criteria=u2 ~= 0
  Dfc_id : Outport  OutDataTypeStr=uint8
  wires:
  Dfc_id_nv/1 -> Bit Clear2/1, Bit Set4/1, Bit Clear1/1
  Bit Set4/1 -> Bit Set/1
  Constant7/1 -> Delay2/1
  Delay2/1 -> Switch2/2
  Switch3/1 -> Switch2/3
  Bit Clear2/1 -> Switch2/1
  Switch2/1 -> Delay3/1, Dfc_id/1
  Bit Set1/1 -> Switch3/1
  Bit Set/1 -> Bit Set1/1
  Switch4/1 -> Switch3/3
  Err/1 -> Switch3/2
  Bit Set2/1 -> Switch4/1
  Bit Clear1/1 -> Bit Set2/1
  Delay3/1 -> Switch4/3
  Heal/1 -> Switch4/2

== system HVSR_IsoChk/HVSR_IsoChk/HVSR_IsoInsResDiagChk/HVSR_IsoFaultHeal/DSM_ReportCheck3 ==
  note: Fault report to diagnostic management system
  Dfc_id_nv : Inport  OutDataTypeStr=uint8
  Err : Inport  Port=2
  Heal : Inport  Port=3
  Bit Clear1 : simulink/Logic and Bit Operations/Bit Clear  iBit=4
  Bit Clear2 : simulink/Logic and Bit Operations/Bit Clear  iBit=3
  Bit Set : simulink/Logic and Bit Operations/Bit Set  iBit=4
  Bit Set1 : simulink/Logic and Bit Operations/Bit Set  iBit=3
  Bit Set2 : simulink/Logic and Bit Operations/Bit Set  iBit=3
  Bit Set4 : simulink/Logic and Bit Operations/Bit Set  iBit=7
  Constant7 : Constant  Value=0  OutDataTypeStr=boolean
  Delay2 : Delay  DelayLength=1  InitialCondition=1
  Delay3 : Delay  DelayLength=1  InitialCondition=0
  Switch2 : Switch  Criteria=u2 ~= 0
  Switch3 : Switch  Criteria=u2 ~= 0
  Switch4 : Switch  Criteria=u2 ~= 0
  Dfc_id : Outport  OutDataTypeStr=uint8
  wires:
  Heal/1 -> Switch4/2
  Delay3/1 -> Switch4/3
  Bit Clear1/1 -> Bit Set2/1
  Bit Set2/1 -> Switch4/1
  Err/1 -> Switch3/2
  Switch4/1 -> Switch3/3
  Bit Set/1 -> Bit Set1/1
  Bit Set1/1 -> Switch3/1
  Switch2/1 -> Dfc_id/1, Delay3/1
  Bit Clear2/1 -> Switch2/1
  Switch3/1 -> Switch2/3
  Delay2/1 -> Switch2/2
  Constant7/1 -> Delay2/1
  Bit Set4/1 -> Bit Set/1
  Dfc_id_nv/1 -> Bit Clear1/1, Bit Set4/1, Bit Clear2/1

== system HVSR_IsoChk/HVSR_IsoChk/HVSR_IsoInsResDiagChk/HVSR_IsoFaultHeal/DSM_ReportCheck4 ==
  note: Fault report to diagnostic management system
  Dfc_id_nv : Inport  OutDataTypeStr=uint8
  Err : Inport  Port=2
  Heal : Inport  Port=3
  Bit Clear1 : simulink/Logic and Bit Operations/Bit Clear  iBit=4
  Bit Clear2 : simulink/Logic and Bit Operations/Bit Clear  iBit=3
  Bit Set : simulink/Logic and Bit Operations/Bit Set  iBit=4
  Bit Set1 : simulink/Logic and Bit Operations/Bit Set  iBit=3
  Bit Set2 : simulink/Logic and Bit Operations/Bit Set  iBit=3
  Bit Set4 : simulink/Logic and Bit Operations/Bit Set  iBit=7
  Constant7 : Constant  Value=0  OutDataTypeStr=boolean
  Delay2 : Delay  DelayLength=1  InitialCondition=1
  Delay3 : Delay  DelayLength=1  InitialCondition=0
  Switch2 : Switch  Criteria=u2 ~= 0
  Switch3 : Switch  Criteria=u2 ~= 0
  Switch4 : Switch  Criteria=u2 ~= 0
  Dfc_id : Outport  OutDataTypeStr=uint8
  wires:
  Dfc_id_nv/1 -> Bit Clear2/1, Bit Set4/1, Bit Clear1/1
  Bit Set4/1 -> Bit Set/1
  Constant7/1 -> Delay2/1
  Delay2/1 -> Switch2/2
  Switch3/1 -> Switch2/3
  Bit Clear2/1 -> Switch2/1
  Switch2/1 -> Delay3/1, Dfc_id/1
  Bit Set1/1 -> Switch3/1
  Bit Set/1 -> Bit Set1/1
  Switch4/1 -> Switch3/3
  Err/1 -> Switch3/2
  Bit Set2/1 -> Switch4/1
  Bit Clear1/1 -> Bit Set2/1
  Delay3/1 -> Switch4/3
  Heal/1 -> Switch4/2

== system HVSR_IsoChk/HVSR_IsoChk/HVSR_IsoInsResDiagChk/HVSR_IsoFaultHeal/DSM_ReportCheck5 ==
  note: Fault report to diagnostic management system
  Dfc_id_nv : Inport  OutDataTypeStr=uint8
  Err : Inport  Port=2
  Heal : Inport  Port=3
  Bit Clear1 : simulink/Logic and Bit Operations/Bit Clear  iBit=4
  Bit Clear2 : simulink/Logic and Bit Operations/Bit Clear  iBit=3
  Bit Set : simulink/Logic and Bit Operations/Bit Set  iBit=4
  Bit Set1 : simulink/Logic and Bit Operations/Bit Set  iBit=3
  Bit Set2 : simulink/Logic and Bit Operations/Bit Set  iBit=3
  Bit Set4 : simulink/Logic and Bit Operations/Bit Set  iBit=7
  Constant7 : Constant  Value=0  OutDataTypeStr=boolean
  Delay2 : Delay  DelayLength=1  InitialCondition=1
  Delay3 : Delay  DelayLength=1  InitialCondition=0
  Switch2 : Switch  Criteria=u2 ~= 0
  Switch3 : Switch  Criteria=u2 ~= 0
  Switch4 : Switch  Criteria=u2 ~= 0
  Dfc_id : Outport  OutDataTypeStr=uint8
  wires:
  Heal/1 -> Switch4/2
  Delay3/1 -> Switch4/3
  Bit Clear1/1 -> Bit Set2/1
  Bit Set2/1 -> Switch4/1
  Err/1 -> Switch3/2
  Switch4/1 -> Switch3/3
  Bit Set/1 -> Bit Set1/1
  Bit Set1/1 -> Switch3/1
  Switch2/1 -> Dfc_id/1, Delay3/1
  Bit Clear2/1 -> Switch2/1
  Switch3/1 -> Switch2/3
  Delay2/1 -> Switch2/2
  Constant7/1 -> Delay2/1
  Bit Set4/1 -> Bit Set/1
  Dfc_id_nv/1 -> Bit Clear1/1, Bit Set4/1, Bit Clear2/1

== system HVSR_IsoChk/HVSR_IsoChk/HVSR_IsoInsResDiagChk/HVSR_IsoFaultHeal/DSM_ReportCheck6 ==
  note: Fault report to diagnostic management system
  Dfc_id_nv : Inport  OutDataTypeStr=uint8
  Err : Inport  Port=2
  Heal : Inport  Port=3
  Bit Clear1 : simulink/Logic and Bit Operations/Bit Clear  iBit=4
  Bit Clear2 : simulink/Logic and Bit Operations/Bit Clear  iBit=3
  Bit Set : simulink/Logic and Bit Operations/Bit Set  iBit=4
  Bit Set1 : simulink/Logic and Bit Operations/Bit Set  iBit=3
  Bit Set2 : simulink/Logic and Bit Operations/Bit Set  iBit=3
  Bit Set4 : simulink/Logic and Bit Operations/Bit Set  iBit=7
  Constant7 : Constant  Value=0  OutDataTypeStr=boolean
  Delay2 : Delay  DelayLength=1  InitialCondition=1
  Delay3 : Delay  DelayLength=1  InitialCondition=0
  Switch2 : Switch  Criteria=u2 ~= 0
  Switch3 : Switch  Criteria=u2 ~= 0
  Switch4 : Switch  Criteria=u2 ~= 0
  Dfc_id : Outport  OutDataTypeStr=uint8
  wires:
  Heal/1 -> Switch4/2
  Delay3/1 -> Switch4/3
  Bit Clear1/1 -> Bit Set2/1
  Bit Set2/1 -> Switch4/1
  Err/1 -> Switch3/2
  Switch4/1 -> Switch3/3
  Bit Set/1 -> Bit Set1/1
  Bit Set1/1 -> Switch3/1
  Switch2/1 -> Dfc_id/1, Delay3/1
  Bit Clear2/1 -> Switch2/1
  Switch3/1 -> Switch2/3
  Delay2/1 -> Switch2/2
  Constant7/1 -> Delay2/1
  Bit Set4/1 -> Bit Set/1
  Dfc_id_nv/1 -> Bit Clear1/1, Bit Set4/1, Bit Clear2/1

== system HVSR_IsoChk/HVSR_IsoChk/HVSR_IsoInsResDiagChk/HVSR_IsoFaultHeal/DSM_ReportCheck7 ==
  note: Fault report to diagnostic management system
  Dfc_id_nv : Inport  OutDataTypeStr=uint8
  Err : Inport  Port=2
  Heal : Inport  Port=3
  Bit Clear1 : simulink/Logic and Bit Operations/Bit Clear  iBit=4
  Bit Clear2 : simulink/Logic and Bit Operations/Bit Clear  iBit=3
  Bit Set : simulink/Logic and Bit Operations/Bit Set  iBit=4
  Bit Set1 : simulink/Logic and Bit Operations/Bit Set  iBit=3
  Bit Set2 : simulink/Logic and Bit Operations/Bit Set  iBit=3
  Bit Set4 : simulink/Logic and Bit Operations/Bit Set  iBit=7
  Constant7 : Constant  Value=0  OutDataTypeStr=boolean
  Delay2 : Delay  DelayLength=1  InitialCondition=1
  Delay3 : Delay  DelayLength=1  InitialCondition=0
  Switch2 : Switch  Criteria=u2 ~= 0
  Switch3 : Switch  Criteria=u2 ~= 0
  Switch4 : Switch  Criteria=u2 ~= 0
  Dfc_id : Outport  OutDataTypeStr=uint8
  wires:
  Heal/1 -> Switch4/2
  Delay3/1 -> Switch4/3
  Bit Clear1/1 -> Bit Set2/1
  Bit Set2/1 -> Switch4/1
  Err/1 -> Switch3/2
  Switch4/1 -> Switch3/3
  Bit Set/1 -> Bit Set1/1
  Bit Set1/1 -> Switch3/1
  Switch2/1 -> Dfc_id/1, Delay3/1
  Bit Clear2/1 -> Switch2/1
  Switch3/1 -> Switch2/3
  Delay2/1 -> Switch2/2
  Constant7/1 -> Delay2/1
  Bit Set4/1 -> Bit Set/1
  Dfc_id_nv/1 -> Bit Clear1/1, Bit Set4/1, Bit Clear2/1

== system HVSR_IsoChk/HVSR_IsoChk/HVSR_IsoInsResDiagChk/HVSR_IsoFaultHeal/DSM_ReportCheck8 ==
  note: Fault report to diagnostic management system
  Dfc_id_nv : Inport  OutDataTypeStr=uint8
  Err : Inport  Port=2
  Heal : Inport  Port=3
  Bit Clear1 : simulink/Logic and Bit Operations/Bit Clear  iBit=4
  Bit Clear2 : simulink/Logic and Bit Operations/Bit Clear  iBit=3
  Bit Set : simulink/Logic and Bit Operations/Bit Set  iBit=4
  Bit Set1 : simulink/Logic and Bit Operations/Bit Set  iBit=3
  Bit Set2 : simulink/Logic and Bit Operations/Bit Set  iBit=3
  Bit Set4 : simulink/Logic and Bit Operations/Bit Set  iBit=7
  Constant7 : Constant  Value=0  OutDataTypeStr=boolean
  Delay2 : Delay  DelayLength=1  InitialCondition=1
  Delay3 : Delay  DelayLength=1  InitialCondition=0
  Switch2 : Switch  Criteria=u2 ~= 0
  Switch3 : Switch  Criteria=u2 ~= 0
  Switch4 : Switch  Criteria=u2 ~= 0
  Dfc_id : Outport  OutDataTypeStr=uint8
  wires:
  Heal/1 -> Switch4/2
  Delay3/1 -> Switch4/3
  Bit Clear1/1 -> Bit Set2/1
  Bit Set2/1 -> Switch4/1
  Err/1 -> Switch3/2
  Switch4/1 -> Switch3/3
  Bit Set/1 -> Bit Set1/1
  Bit Set1/1 -> Switch3/1
  Switch2/1 -> Dfc_id/1, Delay3/1
  Bit Clear2/1 -> Switch2/1
  Switch3/1 -> Switch2/3
  Delay2/1 -> Switch2/2
  Constant7/1 -> Delay2/1
  Bit Set4/1 -> Bit Set/1
  Dfc_id_nv/1 -> Bit Clear1/1, Bit Set4/1, Bit Clear2/1

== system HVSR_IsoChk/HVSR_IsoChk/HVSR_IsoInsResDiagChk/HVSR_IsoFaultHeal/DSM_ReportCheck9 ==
  note: Fault report to diagnostic management system
  Dfc_id_nv : Inport  OutDataTypeStr=uint8
  Err : Inport  Port=2
  Heal : Inport  Port=3
  Bit Clear1 : simulink/Logic and Bit Operations/Bit Clear  iBit=4
  Bit Clear2 : simulink/Logic and Bit Operations/Bit Clear  iBit=3
  Bit Set : simulink/Logic and Bit Operations/Bit Set  iBit=4
  Bit Set1 : simulink/Logic and Bit Operations/Bit Set  iBit=3
  Bit Set2 : simulink/Logic and Bit Operations/Bit Set  iBit=3
  Bit Set4 : simulink/Logic and Bit Operations/Bit Set  iBit=7
  Constant7 : Constant  Value=0  OutDataTypeStr=boolean
  Delay2 : Delay  DelayLength=1  InitialCondition=1
  Delay3 : Delay  DelayLength=1  InitialCondition=0
  Switch2 : Switch  Criteria=u2 ~= 0
  Switch3 : Switch  Criteria=u2 ~= 0
  Switch4 : Switch  Criteria=u2 ~= 0
  Dfc_id : Outport  OutDataTypeStr=uint8
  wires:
  Heal/1 -> Switch4/2
  Delay3/1 -> Switch4/3
  Bit Clear1/1 -> Bit Set2/1
  Bit Set2/1 -> Switch4/1
  Err/1 -> Switch3/2
  Switch4/1 -> Switch3/3
  Bit Set/1 -> Bit Set1/1
  Bit Set1/1 -> Switch3/1
  Switch2/1 -> Dfc_id/1, Delay3/1
  Bit Clear2/1 -> Switch2/1
  Switch3/1 -> Switch2/3
  Delay2/1 -> Switch2/2
  Constant7/1 -> Delay2/1
  Bit Set4/1 -> Bit Set/1
  Dfc_id_nv/1 -> Bit Clear1/1, Bit Set4/1, Bit Clear2/1

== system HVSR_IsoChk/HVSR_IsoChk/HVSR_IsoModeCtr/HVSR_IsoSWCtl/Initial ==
  Enable : EnablePort  StatesWhenEnabling=reset
  Constant2 : Constant  Value=enmSWSta.SWOFF  OutDataTypeStr=Enum: enmSWSta
  Constant3 : Constant  Value=enmSWSta.SWOFF  OutDataTypeStr=Enum: enmSWSta
  Constant6 : Constant  Value=enmSWSta.SWOFF  OutDataTypeStr=Enum: enmSWSta
  Data Type Conversion : DataTypeConversion  OutDataTypeStr=boolean
  Data Type Conversion1 : DataTypeConversion  OutDataTypeStr=boolean
  Data Type Conversion2 : DataTypeConversion  OutDataTypeStr=boolean
  init_bIsoSwt1Ena : Outport  OutDataTypeStr=boolean  InitialOutput=0
  init_bIsoSwt2Ena : Outport  Port=2  OutDataTypeStr=boolean  InitialOutput=0
  init_bIsoSwt3Ena : Outport  Port=3  OutDataTypeStr=boolean  InitialOutput=0
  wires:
  Data Type Conversion2/1 -> init_bIsoSwt1Ena/1
  Data Type Conversion1/1 -> init_bIsoSwt2Ena/1
  Data Type Conversion/1 -> init_bIsoSwt3Ena/1
  Constant3/1 -> Data Type Conversion/1
  Constant6/1 -> Data Type Conversion2/1
  Constant2/1 -> Data Type Conversion1/1

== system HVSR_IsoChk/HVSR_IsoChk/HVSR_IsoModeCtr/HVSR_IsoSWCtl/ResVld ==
  note: 0
  reset_flgVald : Inport
  HVSR_IsoBeginSta : Inport  Port=2
  HVSR_BattInsResVald : Inport  Port=3
  Switch : Switch  Criteria=u2 > Threshold
  HVSR_flgBattInsResVld : Outport
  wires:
  Switch/1 -> HVSR_flgBattInsResVld/1
  HVSR_BattInsResVald/1 -> Switch/3
  HVSR_IsoBeginSta/1 -> Switch/2
  reset_flgVald/1 -> Switch/1

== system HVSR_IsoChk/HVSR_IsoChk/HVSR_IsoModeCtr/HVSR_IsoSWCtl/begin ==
  Enable : EnablePort  StatesWhenEnabling=reset
  Constant3 : Constant  Value=enmSWSta.SWOFF  OutDataTypeStr=Enum: enmSWSta
  Constant5 : Constant  Value=enmSWSta.SWON  OutDataTypeStr=Enum: enmSWSta
  Constant6 : Constant  Value=enmSWSta.SWOFF  OutDataTypeStr=Enum: enmSWSta
  Constant7 : Constant  Value=enmSWSta.SWON  OutDataTypeStr=Enum: enmSWSta
  Data Type Conversion{,1..3} (4 alike) : DataTypeConversion  OutDataTypeStr=boolean
  begin_bIsoSwt1Ena : Outport  OutDataTypeStr=boolean  InitialOutput=0
  begin_bIsoSwt2Ena : Outport  Port=2  OutDataTypeStr=boolean  InitialOutput=0
  begin_bIsoSwt3Ena : Outport  Port=3  OutDataTypeStr=boolean  InitialOutput=0
  reset_flgVald : Outport  Port=4  OutDataTypeStr=boolean  InitialOutput=0
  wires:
  Data Type Conversion3/1 -> begin_bIsoSwt2Ena/1
  Data Type Conversion2/1 -> begin_bIsoSwt1Ena/1
  Data Type Conversion1/1 -> begin_bIsoSwt3Ena/1
  Data Type Conversion/1 -> reset_flgVald/1
  Constant3/1 -> Data Type Conversion/1
  Constant5/1 -> Data Type Conversion1/1
  Constant6/1 -> Data Type Conversion2/1
  Constant7/1 -> Data Type Conversion3/1

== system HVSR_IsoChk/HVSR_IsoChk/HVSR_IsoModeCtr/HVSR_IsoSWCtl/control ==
  Enable : EnablePort  StatesWhenEnabling=reset
  Constant5 : Constant  Value=enmSWSta.SWON  OutDataTypeStr=Enum: enmSWSta
  Constant6 : Constant  Value=enmSWSta.SWOFF  OutDataTypeStr=Enum: enmSWSta
  Constant7 : Constant  Value=enmSWSta.SWON  OutDataTypeStr=Enum: enmSWSta
  Data Type Conversion1 : DataTypeConversion  OutDataTypeStr=boolean
  Data Type Conversion2 : DataTypeConversion  OutDataTypeStr=boolean
  Data Type Conversion3 : DataTypeConversion  OutDataTypeStr=boolean
  ctr_bIsoSwt1Ena : Outport  OutDataTypeStr=boolean  InitialOutput=0
  ctr_bIsoSwt2Ena : Outport  Port=2  OutDataTypeStr=boolean  InitialOutput=0
  ctr_bIsoSwt3Ena : Outport  Port=3  OutDataTypeStr=boolean  InitialOutput=0
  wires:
  Data Type Conversion3/1 -> ctr_bIsoSwt3Ena/1
  Data Type Conversion2/1 -> ctr_bIsoSwt2Ena/1
  Data Type Conversion1/1 -> ctr_bIsoSwt1Ena/1
  Constant5/1 -> Data Type Conversion1/1
  Constant6/1 -> Data Type Conversion2/1
  Constant7/1 -> Data Type Conversion3/1

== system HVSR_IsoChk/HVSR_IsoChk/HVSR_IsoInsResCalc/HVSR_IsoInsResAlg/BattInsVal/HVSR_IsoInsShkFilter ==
  HVSR_flgInsResVld : Inport
  HVSR_resBattInsRes : Inport  Port=2
  Abs1 : Abs
  Constant : Constant  Value=0  OutDataTypeStr=boolean
  Constant1 : Constant  Value=HVSR_tiTaskTime_C
  Constant2 : Constant  Value=HVSR_numCycleTimeCnt_C
  Constant3 : Constant  Value=single(0)
  Constant4 : Constant  Value=HVSR_deltInsRes_C
  Constant5 : Constant  Value=single(0.01)
  Delay2 : Delay  DelayLength=1  InitialCondition=0
  Delay3 : Delay  DelayLength=1  InitialCondition=0
  EdgeRising : Subsystem  TreatAsAtomicUnit=on  RTWFcnName=EdgeRising  RTWFileName=SrvLib
  EdgeRising1 : Subsystem  TreatAsAtomicUnit=on  RTWFcnName=EdgeRising  RTWFileName=SrvLib
  EdgeRising2 : Subsystem  TreatAsAtomicUnit=on  RTWFcnName=EdgeRising  RTWFileName=SrvLib
  EdgeRising3 : Subsystem  TreatAsAtomicUnit=on  RTWFcnName=EdgeRising  RTWFileName=SrvLib
  Gain : Gain  Gain=single(1000)
  Logical Operator : Logic  Operator=NOT  AllPortsSameDT=off  OutDataTypeStr=boolean
  Logical Operator1 : Logic  Operator=OR  AllPortsSameDT=off  OutDataTypeStr=boolean
  RS_FlipFlop : Subsystem
  Relational Operator1 : RelationalOperator  OutDataTypeStr=boolean  RndMeth=Simplest
  Relational Operator2 : RelationalOperator  Operator=>  OutDataTypeStr=boolean  RndMeth=Simplest
  Subsystem2 : Subsystem
  Subsystem3 : Subsystem
  Subtract1 : Sum  Inputs=+-
  Subtract2 : Sum  Inputs=+-
  Terminator : Terminator
  Timer2 : Subsystem
  HVSR_flgInsResChngVld : Outport
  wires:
  Abs1/1 -> Relational Operator1/1
  Subtract1/1 -> Abs1/1
  Constant1/1 -> Timer2/2(Ts)
  HVSR_flgInsResVld/1 -> EdgeRising2/1(u), EdgeRising1/1(u)
  Subsystem3/1(Q) -> Timer2/1(En), Logical Operator/1
  Relational Operator1/1 -> Subsystem3/1(set)
  Subsystem2/1(Out1) -> Subtract1/1, Delay3/1
  Constant4/1 -> Gain/1
  Relational Operator2/1 -> Delay2/1
  Timer2/1(Timer) -> Relational Operator2/1
  Constant2/1 -> Subtract2/1
  HVSR_resBattInsRes/1 -> Subsystem2/1(In1)
  EdgeRising1/1(y) -> Subsystem2/Enable
  Delay2/1 -> Subsystem3/2(clear), EdgeRising/1(u)
  EdgeRising/1(y) -> Timer2/3(Rst)
  Constant3/1 -> Timer2/4(Vst)
  Logical Operator/1 -> Logical Operator1/2
  Subtract2/1 -> Relational Operator2/2
  Constant5/1 -> Subtract2/2
  Gain/1 -> Relational Operator1/2
  EdgeRising3/1(y) -> Logical Operator1/1  "HVSR_flgIFlipFlopVal"
  Logical Operator1/1 -> HVSR_flgInsResChngVld/1  "HVSR_flgInsResChngVld"
  EdgeRising2/1(y) -> RS_FlipFlop/1(S)
  RS_FlipFlop/1(Q) -> EdgeRising3/1(u)
  Constant/1 -> RS_FlipFlop/2(R)
  RS_FlipFlop/2(!Q) -> Terminator/1
  Delay3/1 -> Subtract1/2
